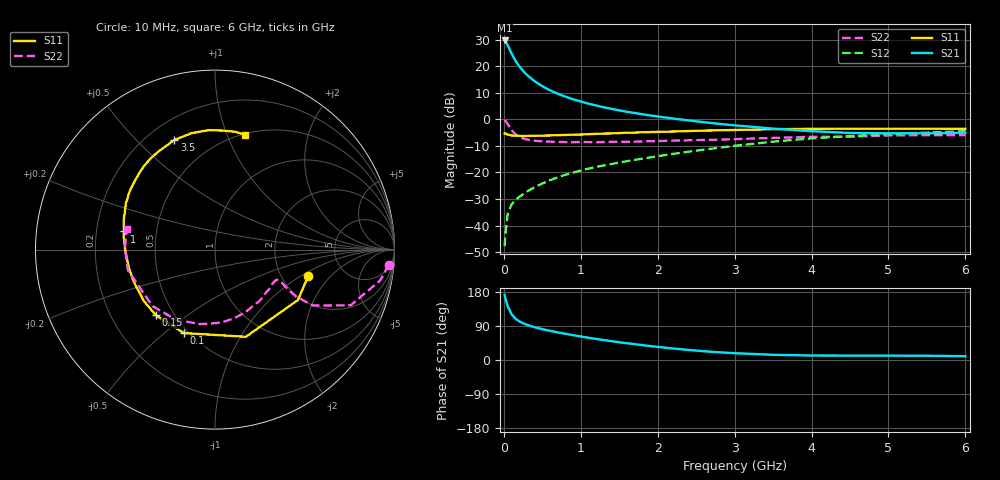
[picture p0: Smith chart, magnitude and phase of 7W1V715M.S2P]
! Infineon Technologies  Discrete & RF Semiconductors
! BFS17W
! Si NPN RF Bipolar Junction Transistor in SOT323
! VCE = 1.75 V  IC = 15 mA
! Common Emitter S-Parameters:  August  1999
# GHz  S  MA  R  50
!  f  S11  S21  S12  S22
! GHz  MAG  ANG  MAG  ANG  MAG  ANG  MAG  ANG
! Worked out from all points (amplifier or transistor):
!   36 points, 10 MHz to 6 GHz, reference 50 ohm
!   highest |S21| = 29.7 dB at 10 MHz (marker M1)
!   |S21| within 3 dB of that: start of sweep to 69.67 MHz
!   unconditionally stable (mu >= 1): 289.1 MHz to 2.998 GHz; 3.903 GHz to end of sweep
!   at 250 MHz: K = 0.95, MSG = 23.2 dB, |S12| = -28.2 dB
!   at 1.4 GHz: K = 1.24, MAG = 7.4 dB, |S12| = -16.8 dB
!   at 6 GHz: K = 1.09, MAG = -2.1 dB, |S12| = -4.5 dB
!   S11 on the Smith chart (normalised r, x): 10 MHz: 2.80, -1.17; 100 MHz: 0.47, -0.58; 150 MHz: 0.40, -0.39; 1 GHz: 0.32, +0.09; 3.5 GHz: 0.31, +0.65; 6 GHz: 0.51, +1.16
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0.01  0.5395 -15.9  30.48 171.7  0.0041 77.7  0.9724 -5.0
0.02  0.5409 -31.3  29.54 163.0  0.0067 82.2  0.9359 -10.6
0.05  0.5152 -70.5  24.87 141.8  0.0167 64.5  0.8176 -22.3
0.1  0.4962 -110.4  17.34 121.0  0.0249 55.9  0.6283 -29.7
0.15  0.4923 -131.9  12.75 109.3  0.0304 53.2  0.5235 -30.1
0.2  0.4891 -144.1  9.983 102.2  0.0347 55.6  0.4691 -28.8
0.25  0.4845 -152.8  8.14 96.9  0.0387 56.4  0.4356 -27.4
0.3  0.4867 -158.8  6.859 92.9  0.0437 59.0  0.4178 -26.5
0.4  0.4901 -167.5  5.217 86.4  0.0527 61.4  0.3944 -25.6
0.5  0.4926 -173.5  4.204 81.4  0.0618 63.1  0.3857 -25.8
0.6  0.497 -177.8  3.514 77.0  0.0715 64.6  0.3796 -26.7
0.7  0.503 178.2  3.034 72.9  0.0809 65.6  0.3754 -28.4
0.8  0.5074 174.6  2.671 69.1  0.0903 65.8  0.3726 -30.5
1  0.5167 168.7  2.161 62.2  0.1089 66.6  0.3745 -34.8
1.1  0.5258 165.4  1.972 58.7  0.118 66.3  0.3727 -37.9
1.6  0.5601 152.5  1.387 44.2  0.163 66.4  0.3771 -53.3
2.2  0.5897 138.7  1.035 30.4  0.2234 65.4  0.3966 -73.9
2.8  0.6217 125.1  0.822 20.3  0.2919 62.1  0.4148 -95.1
3.5  0.6513 110.4  0.668 13.7  0.3801 55.4  0.4472 -119.4
4.5  0.6666 92.7  0.553 11.5  0.4817 42.4  0.4705 -153.5
5.5  0.666 80.1  0.545 11.2  0.5634 30.5  0.5013 179.2
6  0.6614 75.3  0.558 10.0  0.5967 24.7  0.5045 167.1
